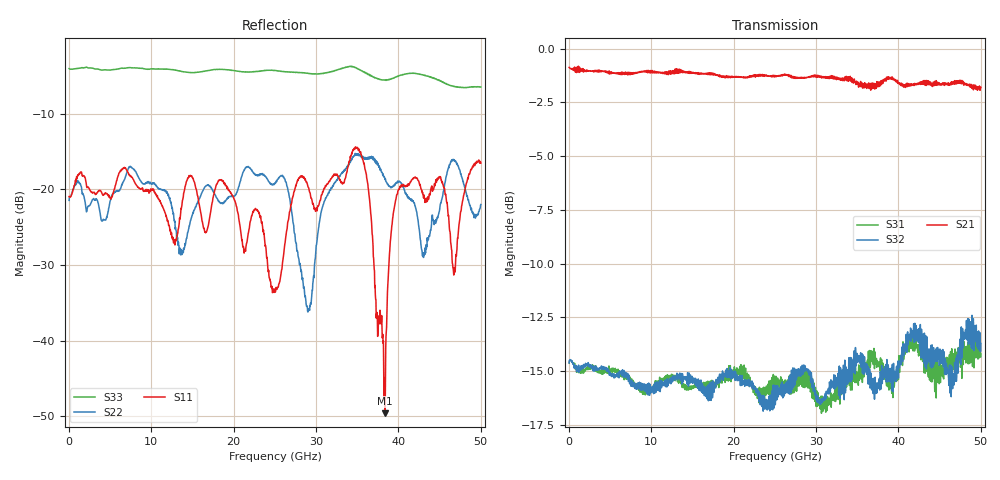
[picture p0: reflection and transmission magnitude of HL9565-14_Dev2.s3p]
! 1/5/2021 8:31:18 AM
! H:\PRODUCTION_DATA\TEMP_S3P.S3P
! CHANNEL.1
! TR.MEASUREMENT
! CORRECTED.DATA
# GHZ S RI R 50.0
! FREQ.GHZ  S11RE  S11IM  S12RE  S12IM  S13RE  S13IM
!  S21RE  S21IM  S22RE  S22IM  S23RE  S23IM
!  S31RE  S31IM  S32RE  S32IM  S33RE  S33IM
!; PortSelection: Port_123
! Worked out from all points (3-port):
!   1429 points, 35 MHz to 50.02 GHz, reference 50 ohm
!   strongest paths, dB at 35 MHz, 12.53 GHz, 25.02 GHz, 37.52 GHz, 50.02 GHz:
!     S21: -0.9, -1.1, -1.3, -1.7, -1.8
!     S32: -14.6, -15.5, -16.0, -15.5, -13.7
!     S31: -14.6, -15.5, -15.5, -14.6, -14.2
!   lowest |S11| = -49.6 dB at 38.4 GHz (marker M1), VSWR 1.01, Z = 49.8 + j0.222 ohm
!   |S11| at or under -10 dB: start of sweep to end of sweep
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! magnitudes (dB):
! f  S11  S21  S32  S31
! 35 MHz  -20.9  -0.9  -14.6  -14.6
! 18.52 GHz  -18.7  -1.3  -15.2  -15.4
! 25.02 GHz  -33.3  -1.3  -16.0  -15.5
! 29.09 GHz  -19.7  -1.3  -14.9  -15.1
! 35 GHz  -14.4  -1.7  -14.6  -15.2
! 38.4 GHz  -49.6  -1.4  -15.3  -15.4
! 40.04 GHz  -20.0  -1.6  -14.7  -14.8
! 43.05 GHz  -21.1  -1.6  -14.3  -14.0
! 46.76 GHz  -30.5  -1.6  -15.6  -14.9
! 50.02 GHz  -16.5  -1.8  -13.7  -14.2
